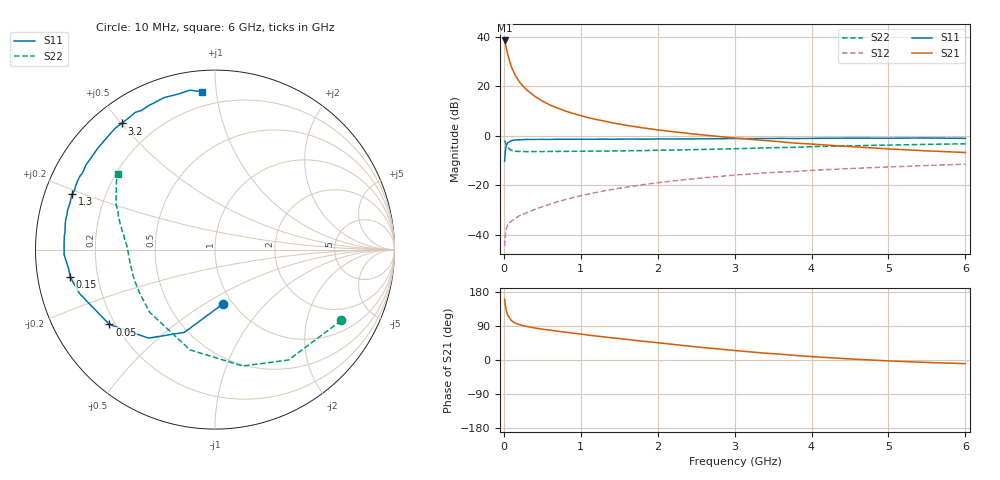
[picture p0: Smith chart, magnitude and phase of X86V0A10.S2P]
! SIEMENS Small Signal Semiconductors
! BFP136W
! Si NPN RF Bipolar Junction Transistor in SOT343
! VCE = 6 V  IC = 100 mA
! Common Emitter S-Parameters:  September  1994
# GHz  S  MA  R  50
!  f  S11  S21  S12  S22
! GHz  MAG  ANG  MAG  ANG  MAG  ANG  MAG  ANG
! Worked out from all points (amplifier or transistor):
!   40 points, 10 MHz to 6 GHz, reference 50 ohm
!   highest |S21| = 38.4 dB at 10 MHz (marker M1)
!   |S21| within 3 dB of that: start of sweep to 31.59 MHz
!   unconditionally stable (mu >= 1): 575.3 MHz to 2.948 GHz
!   at 200 MHz: K = 0.66, MSG = 27.1 dB, |S12| = -32.3 dB
!   at 1.5 GHz: K = 1.10, MAG = 11.0 dB, |S12| = -21.2 dB
!   at 6 GHz: K = 0.97, MSG = 2.4 dB, |S12| = -11.5 dB
!   S11 on the Smith chart (normalised r, x): 10 MHz: 0.90, -0.60; 50 MHz: 0.18, -0.31; 150 MHz: 0.10, -0.09; 1.3 GHz: 0.08, +0.19; 3.2 GHz: 0.08, +0.50; 6 GHz: 0.11, +0.91
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0.01  0.3071 -82.1  83.5 160.4  0.0059 68.5  0.8065 -29.3
0.02  0.4915 -110.3  71.77 144.1  0.01 57.9  0.7392 -56.3
0.03  0.6168 -126.9  60.72 132.4  0.0129 49.2  0.6668 -76.6
0.05  0.7212 -144.7  43.4 118.3  0.0161 39.1  0.5758 -104.0
0.1  0.7939 -162.1  24.05 103.7  0.0189 36.3  0.5043 -136.2
0.15  0.8208 -169.2  16.39 97.4  0.0214 38.3  0.4852 -149.6
0.2  0.8232 -172.9  12.32 93.5  0.0242 39.9  0.4802 -157.1
0.25  0.834 -176.2  9.948 90.6  0.026 42.7  0.4794 -161.8
0.3  0.841 -178.0  8.316 88.4  0.028 45.0  0.4774 -164.9
0.4  0.8413 178.1  6.268 84.6  0.0325 48.7  0.4786 -169.2
0.5  0.843 175.1  4.998 81.4  0.037 51.4  0.4794 -172.1
0.6  0.8418 173.1  4.168 78.8  0.0413 53.6  0.4803 -174.1
0.7  0.8462 170.5  3.596 75.8  0.0467 55.8  0.4819 -175.5
0.9  0.8475 166.8  2.815 70.9  0.0563 57.6  0.4836 -178.2
1.1  0.8484 162.4  2.302 65.5  0.0663 58.4  0.4875 -179.9
1.3  0.8539 158.7  1.978 60.9  0.0768 58.6  0.4907 178.4
1.7  0.8566 151.6  1.526 51.8  0.097 57.1  0.4984 175.3
2.2  0.8593 143.3  1.203 41.2  0.1221 53.9  0.512 171.7
3.2  0.8747 126.5  0.845 21.5  0.1685 45.0  0.5557 163.1
4.5  0.8933 108.4  0.602 2.8  0.2173 33.7  0.6254 151.8
5.5  0.8992 99.0  0.494 -6.4  0.2501 25.6  0.6687 145.2
6  0.8831 94.7  0.458 -9.6  0.2663 21.4  0.6846 142.3
